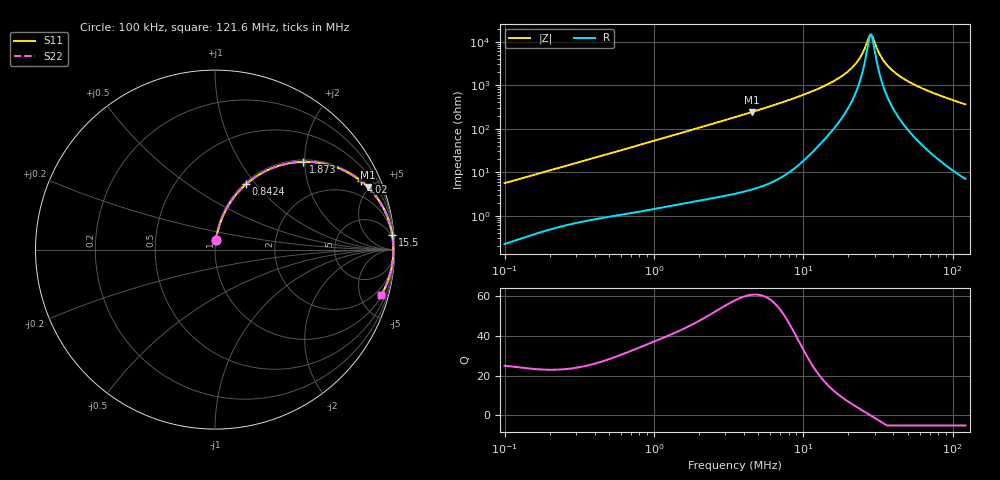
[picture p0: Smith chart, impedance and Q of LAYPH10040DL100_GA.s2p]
! LAYPH10040DL100_GA  S-PARAMETER MODEL  ( General Type )
! Model Generated by TAIYO YUDEN Corporation (http://www.ty-top.com)
! Version 1.0
! TAIYO YUDEN Control No. 180920NI43SB-FBB
! Copyright(c) 2018 TAIYO YUDEN CO.,LTD. All Rights Reserved.
! Product Description (link to TY-COMPAS)
! https://ds.yuden.co.jp/TYCOMPAS/or/detail?pn=LAYPH10040DL100MGA&u=M
! Products Name : Inductors
! Characteristics :
!  Inductance : 10 uH , SRF(min) : -Hz , DC Resistance(max) : 0.035 Ohm
!  Rated Current : Saturation :3.7 A , Temp Rise : 2 A (25 degC)
!  Case Size : 10.1 x 10.0 / 0.398 x 0.394 [mm/inch] , Thickness : 4 / 0.157 [mm/inch]
!  (Conditions: Temperature = 25 degC , DC Bias Current/Voltage = 0A / 0V)
! External Node Assignments :
!  1  o---GGG---o  2
! GND o---------o GND
! Frequency Range : 0.1MHz  -  121.638923MHz  [ 402 STEP ]
# MHz S RI R 50
! Freq[MHz].  S11 Real  S11 Imag  S21 Real  S21 Imag  S12 Real  S12 Imag  S22 Real  S22 Imag
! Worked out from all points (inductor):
!   401 points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, 100 kHz to 121.6 MHz, reference 50 ohm
!   read as one part in series: L = 8.85 uH near 103.6 kHz
!   highest Q = 60.4 at 4.552 MHz (marker M1), where L = 8.49 uH
!   self-resonance near 27.86 MHz
!   S11 on the Smith chart (normalised r, x): 100 kHz: 1.00, +0.11; 842.4 kHz: 1.03, +0.89; 1.873 MHz: 1.04, +1.96; 4.02 MHz: 1.07, +4.26; 15.5 MHz: 3, +23; 121.6 MHz: 1.14, -7.26
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0.1  0.00535 0.0556  0.9946 -0.0556  0.9946 -0.0556  0.00535 0.0556
0.328662  0.037 0.1694  0.963 -0.1694  0.963 -0.1694  0.037 0.1694
0.842407  0.1724 0.3636  0.8276 -0.3636  0.8276 -0.3636  0.1724 0.3636
1.080188  0.2503 0.4202  0.7497 -0.4202  0.7497 -0.4202  0.2503 0.4202
1.873236  0.4914 0.4892  0.5086 -0.4892  0.5086 -0.4892  0.4914 0.4892
3.550168  0.7746 0.4093  0.2254 -0.4093  0.2254 -0.4093  0.7746 0.4093
4.020108  0.8157 0.3794  0.1843 -0.3794  0.1843 -0.3794  0.8157 0.3794
4.552254  0.851 0.3479  0.149 -0.3479  0.149 -0.3479  0.851 0.3479
6.971574  0.9335 0.2399  0.0665 -0.2399  0.0665 -0.2399  0.9335 0.2399
11.46267  0.9761 0.1342  0.0239 -0.1342  0.0239 -0.1342  0.9761 0.1342
15.50249  0.9866 0.0835  0.0134 -0.0835  0.0134 -0.0835  0.9866 0.0835
18.84695  0.9902 0.0548  0.00976 -0.0548  0.00976 -0.0548  0.9902 0.0548
22.11338  0.9921 0.0327  0.00792 -0.0327  0.00792 -0.0327  0.9921 0.0327
24.16677  0.9927 0.0209  0.00728 -0.0209  0.00728 -0.0209  0.9927 0.0209
27.36575  0.9932 0.00445  0.00683 -0.00445  0.00683 -0.00445  0.9932 0.00445
28.3552  0.9932 -0.000232  0.00679 0.000232  0.00679 0.000232  0.9932 -0.000232
29.38042  0.9932 -0.00491  0.00679 0.00491  0.00679 0.00491  0.9932 -0.00491
33.26954  0.9929 -0.0214  0.00713 0.0214  0.00713 0.0214  0.9929 -0.0214
37.67347  0.992 -0.0382  0.00801 0.0382  0.00801 0.0382  0.992 -0.0382
44.99481  0.9896 -0.0633  0.0104 0.0633  0.0104 0.0633  0.9896 -0.0633
57.69523  0.9835 -0.1017  0.0165 0.1017  0.0165 0.1017  0.9835 -0.1017
121.6389  0.9252 -0.2536  0.0748 0.2536  0.0748 0.2536  0.9252 -0.2536
